TYPE ST_RECIPE :
STRUCT
	// L2N
	timeMachine1 : TIME;
	timeMachine2 : TIME;
	directionMachine1 : BOOL;
	directionMachine2 : BOOL;
	
	// RR
	positionSequence : ARRAY [0..9] OF ST_POSITION;
END_STRUCT
END_TYPE
